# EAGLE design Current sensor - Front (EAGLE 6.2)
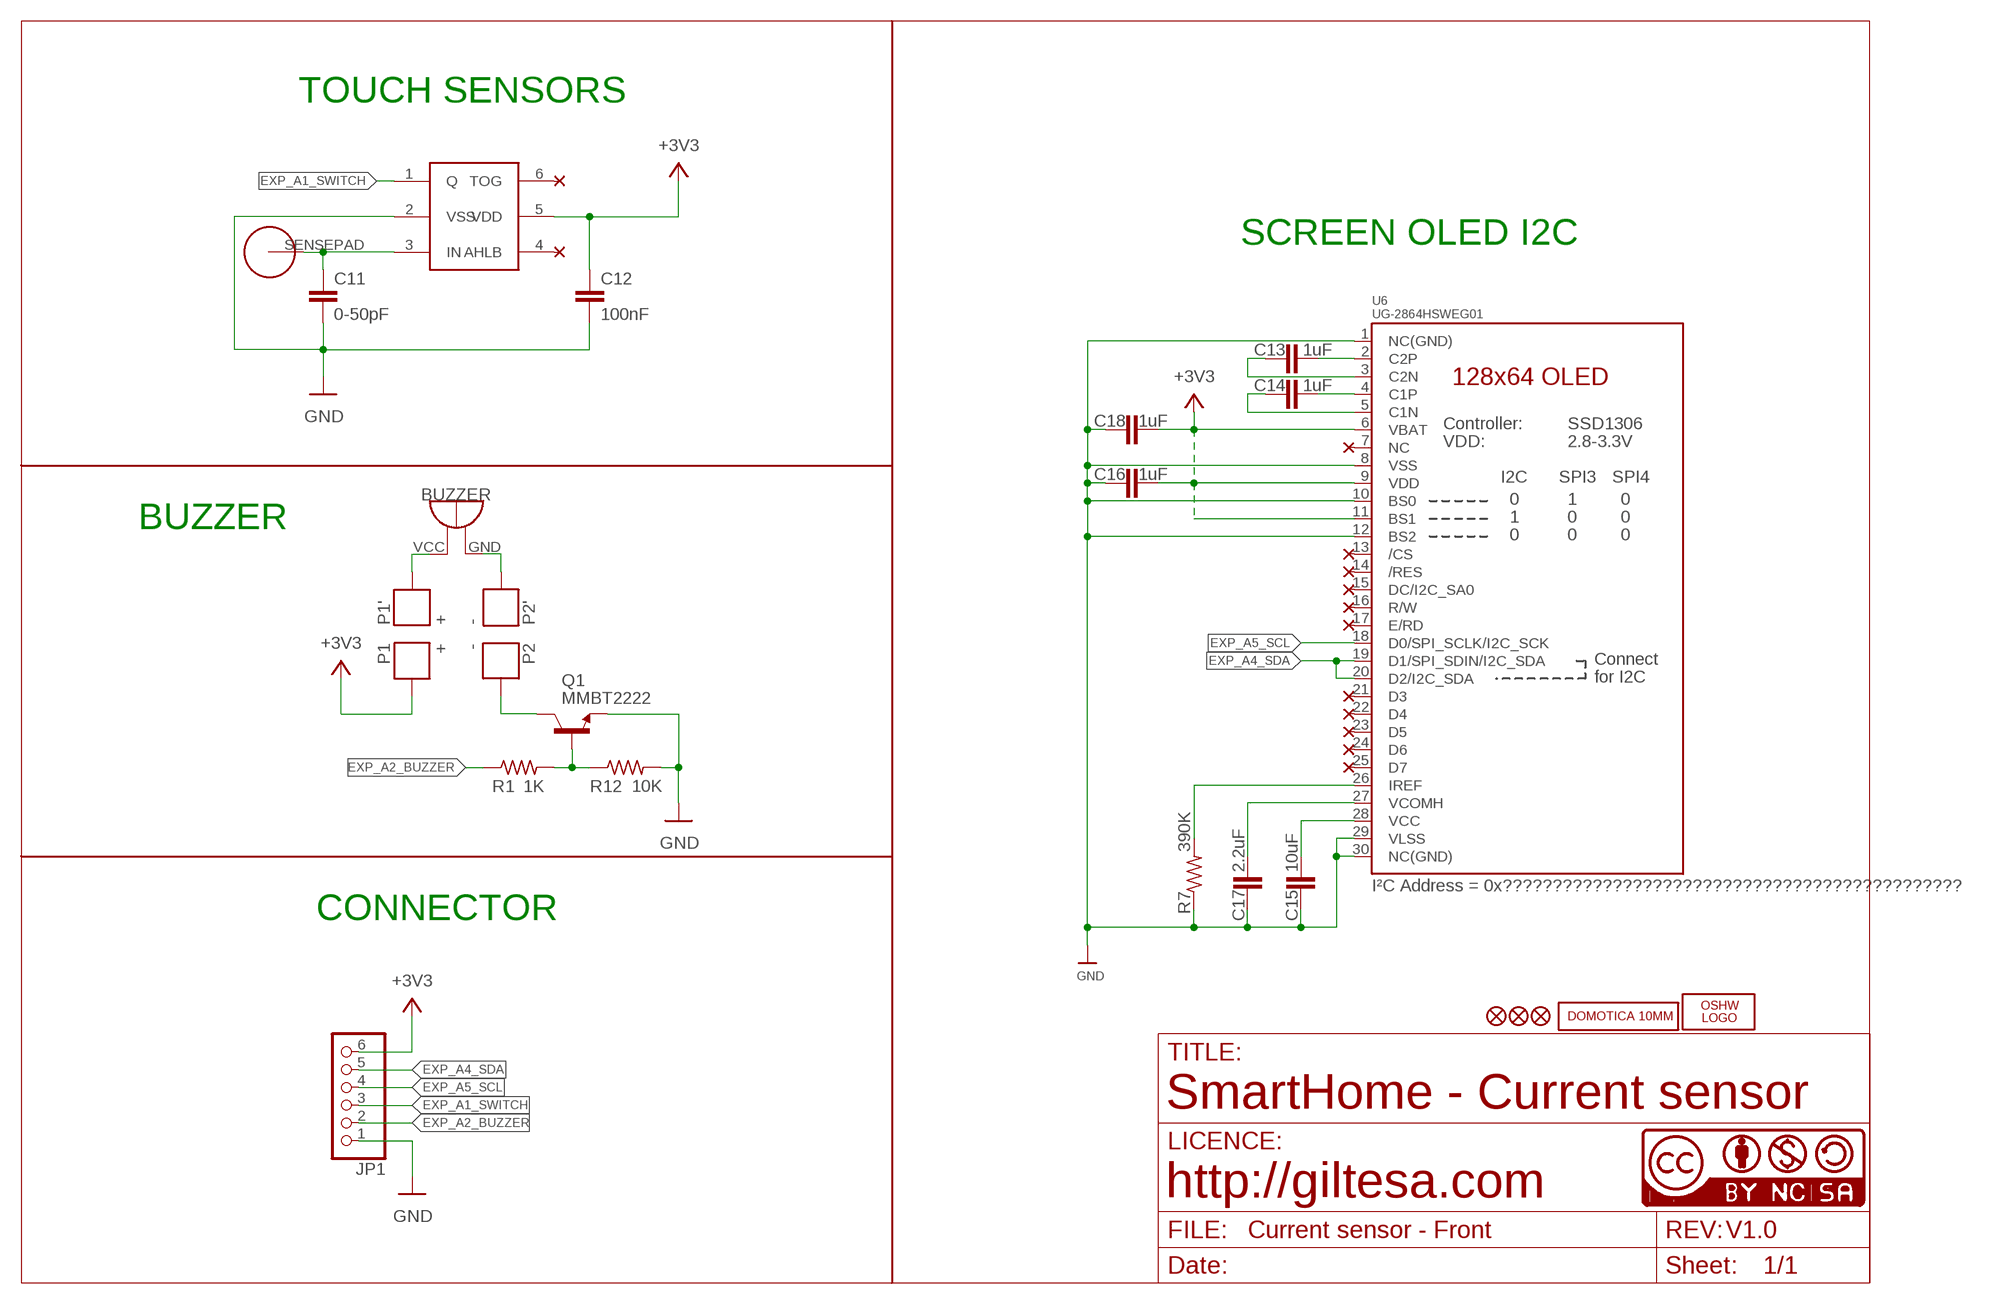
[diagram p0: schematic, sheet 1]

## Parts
BUZZER  BUZZER_9MM  [BUZZER_9MM]
C11  0-50pF  C0603  [C0603]
C12  100nF  C0603  [C0603]
C13  1uF  C0603  [C0603]
C14  1uF  C0603  [C0603]
C15  10uF  C0805  [C0805]
C16  1uF  C0603  [C0603]
C17  2.2uF  C0805  [C0805]
C18  1uF  C0603  [C0603]
JP1  PINHD-1X6B  [1X06-BIG]
LOGO1  OSHW_LOGO_FILLX0150-NT  [OSHW_FILLX150_NOTEXT]
P1  +  1X01_SMT_1.8MM  [1X01_SMT_1.8MM]
P1'  +  1X01_SMD_0.5MM  [1X01_SMD_0.5MM]
P2  -  1X01_SMT_1.8MM  [1X01_SMT_1.8MM]
P2'  -  1X01_SMD_0.5MM  [1X01_SMD_0.5MM]
Q1  MMBT2222  TRANSISTOR_NPNSOT23  [SOT23]
R1  1K  R0603  [R0603]
R7  390K  R0805  [R0805]
R12  10K  R0603  [R0603]
TTP1  TTP223  TTP223-BA6  [SOT-23-6]
U6  UG-2864HSWEG01  DISP_OLED_UG-2864HSWEG010.96"_2  [UG-2864HSWEG01_0.96IN_WRAPAROUND_2]
U$5  DOMOTICA-10MM  [DOMOTICA-10MM]
U$6  FIDUCIAL1X2  [FIDUCIAL-1X2]
U$7  FIDUCIAL1X2  [FIDUCIAL-1X2]
U$10  HTTM_SENSEPAD_NO_MARK  [HTTM_SENSEPAD_NO_MARK]
U$14  FIDUCIAL1X2  [FIDUCIAL-1X2]
U$20  CC-NC-BCNIX  [CC-NC-B_NIX]

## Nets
+3V3: C12.1 C16.2 C18.2 JP1.6 P1.P$1 TTP1.5(VDD) U6.6(VBAT) U6.9(VDD) U6.11(BS1)
EXP_A1_SWITCH: JP1.3 TTP1.1(Q)
EXP_A2_BUZZER: JP1.2 R1.1
EXP_A4_SDA: JP1.5 U6.19(D1/SPI_SDIN/I2C_SDA) U6.20(D2/I2C_SDA)
EXP_A5_SCL: JP1.4 U6.18(D0/SPI_SCLK/I2C_SCK)
GND: C11.2 C12.2 C15.1 C16.1 C17.1 C18.1 JP1.1 Q1.2(E) R7.1 R12.2 TTP1.2(VSS) U6.1(NC(GND)) U6.8(VSS) U6.10(BS0) U6.12(BS2) U6.29(VLSS) U6.30(NC(GND))
N$1: BUZZER.VCC P1'.P$1
N$2: BUZZER.GND P2'.P$1
N$3: P2.P$1 Q1.3(C)
N$6: Q1.1(B) R1.2 R12.1
N$8: C15.2 U6.28(VCC)
N$9: C17.2 U6.27(VCOMH)
N$10: C13.2 U6.2(C2P)
N$11: C13.1 U6.3(C2N)
N$13: C11.1 TTP1.3(IN) U$10.SENSEPAD
N$14: C14.2 U6.4(C1P)
N$15: C14.1 U6.5(C1N)
N$16: R7.2 U6.26(IREF)
Unconnected: TTP1.4(AHLB) TTP1.6(TOG) U6.7(NC) U6.13(/CS) U6.14(/RES) U6.15(DC/I2C_SA0) U6.16(R/W) U6.17(E/RD) U6.21(D3) U6.22(D4) U6.23(D5) U6.24(D6) U6.25(D7)

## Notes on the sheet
- TOUCH SENSORS
- SCREEN OLED I2C
- BUZZER
- I²C Address = 0x??????????????????????????????????????????????
- CONNECTOR
- SmartHome - Current sensor
- http://giltesa.com
- V1.0

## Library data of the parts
BUZZER = ,giltesa:BUZZER
C11-C14 C16 C18 = ,giltesa:C0603
C15 C17 = ,giltesa:C0805
JP1 = adafruit:PINHD-1X6: PIN HEADER
LOGO1 = ohw-logo:OSHW_LOGO_FILL
P1 P1' P2 P2' = ,giltesa:1X01
Q1 = SparkFun:TRANSISTOR_NPN: Transistor NPN BJT configuration in SOT23 package. MMBT2222 is the common NPN we use. Double check BCE configuration again layout.
R1 R12 = ,giltesa:R0603
R7 = ,giltesa:R0805
TTP1 = NCA_Sensors:TTP223-BA6: TTP223 touch sensor
U6 = microbuilder:DISP_OLED_UG-2864HSWEG01: UG-2864HSWEG01 OLED display Both 1.3" and 0.96" models share the same FPC tab footprint, only the screen dimensions vary.
U$5 = ,giltesa_logos:DOMOTICA-10MM
U$6 U$7 U$14 = SparkFun:FIDUCIAL: Fiducial Alignment Points
U$10 = ,giltesa:HTTM_SENSEPAD
U$20 = cc-by-nc-sa:CC-NC-BC: All hardware is licensed under the Creative Commons

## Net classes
2 gnd: width 0.305 mm, drill 0.406 mm, clearance 0.203 mm
3 usbvcc: width 0.203 mm, drill 0.406 mm, clearance 0.203 mm
4 USBpair: width 0.254 mm, drill 0.406 mm, clearance 0.61 mm

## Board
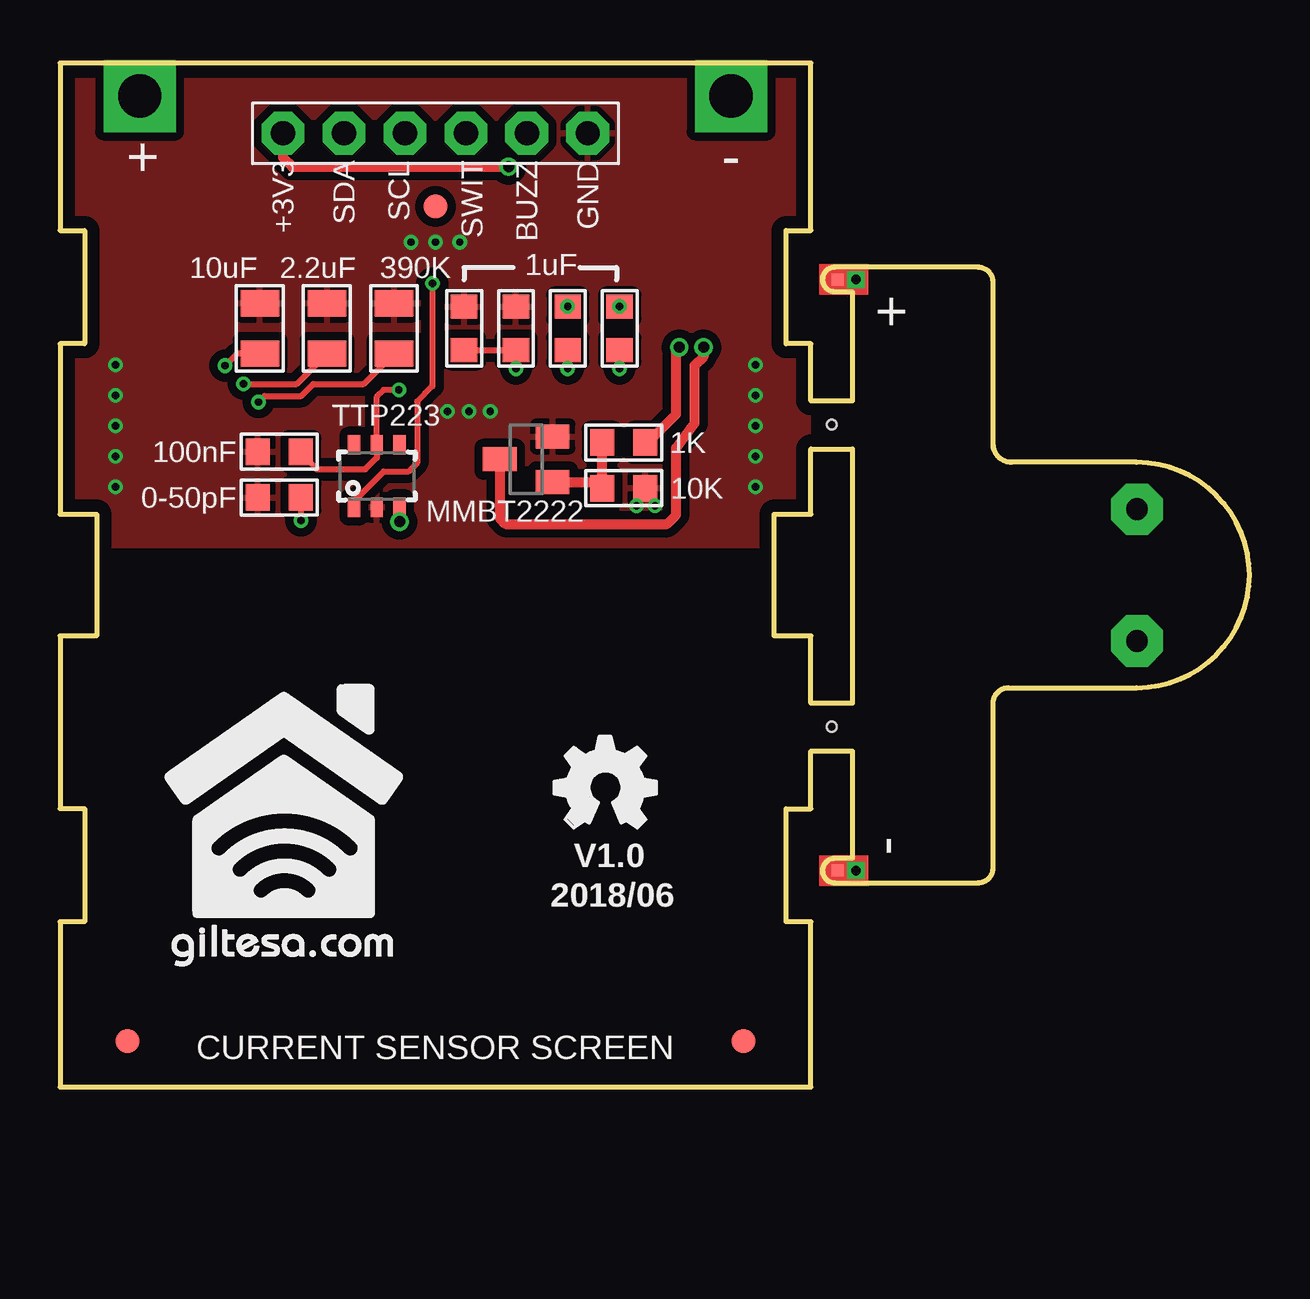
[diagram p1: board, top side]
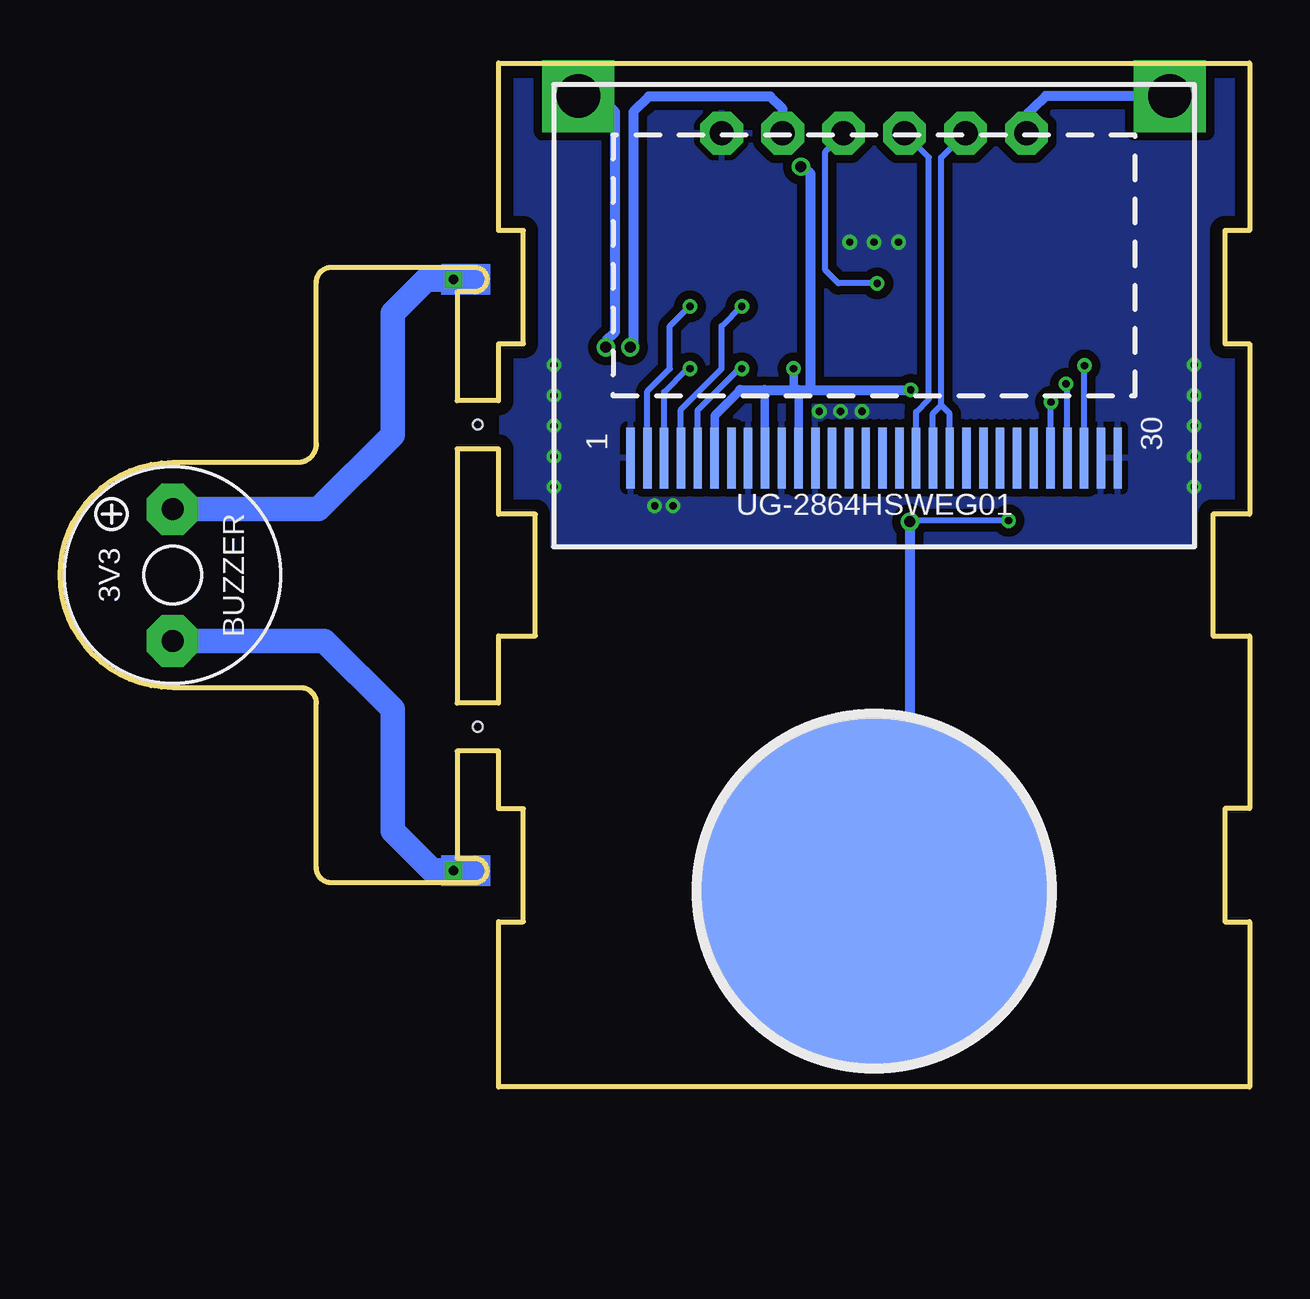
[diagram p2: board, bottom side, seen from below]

Size 49.56 x 42.67 mm. Coordinates in mm from the lower left corner, seen from the top.
Outline: 0,0 31.28,0 31.28,6.88 30.26,6.88 30.26,11.59 31.28,11.59 31.28,13.99 33.02,13.99 33.02,9.53 32.28,9.53 arc180 32.28,8.51 38.25,8.51 arc90 38.88,9.14 38.88,16 arc-90 39.52,16.64 44.86,16.64 arc180 44.86,26.04 39.64,26.04 arc-90 38.88,26.8 38.88,33.53 arc90 38.25,34.16 32.28,34.16 arc180 32.28,33.15 33.02,33.15 33.02,28.6 31.28,28.6 31.28,30.97 30.26,30.97 30.26,35.69 31.28,35.69 31.28,42.67 0,42.67 0,35.69 1.03,35.69 1.03,30.98 0,30.98 0,23.88 1.52,23.88 1.52,18.8 0,18.8 0,11.6 1.03,11.6 1.03,6.88 0,6.88 0,0
Outline: 31.28,16 31.28,18.8 29.76,18.8 29.76,23.88 31.28,23.88 31.28,26.59 33.02,26.59 33.02,16 31.28,16
Copper layers (1*16): Top 0.035mm / dielectric 1.6mm / Bottom 0.035mm
Design rules: minimum track width 6mil, minimum drill 12mil, track to track 6mil, track to pad 6mil, pad to pad 6mil, via to via 8mil, smd to smd 0mil, copper to edge 20mil, drill to drill 10mil, minimum pad ring 6mil, minimum via ring 6mil, stop-mask expansion 0mil, vias tented up to drill 100mil, thermal gap 10mil
Holes 0.41 mm at 32.15,27.61 32.15,15.01
tRestrict: area 31.6,8.1 to 33.7,34.5
bRestrict: area 31.6,8.1 to 33.7,34.5

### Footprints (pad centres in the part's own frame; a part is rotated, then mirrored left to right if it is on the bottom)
BUZZER_9MM = drill 0.914 pad 2.159 octagon: GND -2.743,0; VCC 2.743,0
C0603 = smd 1 x 1.1: 1 -0.901,0; 2 0.901,0
C0805 = smd 1.1 x 1.6: 1 -1.05,0; 2 1.05,0
1X06-BIG = drill 1.016 pad 1.778 octagon: 1 -6.35,0; 2 -3.81,0; 3 -1.27,0; 4 1.27,0; 5 3.81,0; 6 6.35,0
1X01_SMT_1.8MM = drill 1.8 pad 3 square: P$1 0,0
1X01_SMD_0.5MM = smd 0.5 x 0.5: P$1 0,0
SOT23 = smd 1 x 1.4: 1 -0.95,-1.1; 2 0.95,-1.1; 3 0,1.1
R0603 = smd 1 x 1.1: 1 -0.901,0; 2 0.901,0
R0805 = smd 1.1 x 1.6: 1 -1.05,0; 2 1.05,0
SOT-23-6 = smd 0.51 x 0.8: 1 0.955,-0.03; 2 1.905,-0.03; 3 2.855,-0.03; 4 2.855,2.57; 5 1.905,2.57; 6 0.955,2.57
UG-2864HSWEG01_0.96IN_WRAPAROUND_2 = smd 0.35 x 2.54 bottom: 1 10.15,-1.2; 2 9.45,-1.2; 3 8.75,-1.2; 4 8.05,-1.2; 5 7.35,-1.2; 6 6.65,-1.2; 7 5.95,-1.2; 8 5.25,-1.2; 9 4.55,-1.2; 10 3.85,-1.2; 11 3.15,-1.2; 12 2.45,-1.2; 13 1.75,-1.2; 14 1.05,-1.2; 15 0.35,-1.2; 16 -0.35,-1.2; 17 -1.05,-1.2; 18 -1.75,-1.2; 19 -2.45,-1.2; 20 -3.15,-1.2; 21 -3.85,-1.2; 22 -4.55,-1.2; 23 -5.25,-1.2; 24 -5.95,-1.2; 25 -6.65,-1.2; 26 -7.35,-1.2; 27 -8.05,-1.2; 28 -8.75,-1.2; 29 -9.45,-1.2; 30 -10.15,-1.2
FIDUCIAL-1X2 = smd 1 x 1: 1 0,0
HTTM_SENSEPAD_NO_MARK = smd 14.5 x 14.5: SENSEPAD -0.001,0.001

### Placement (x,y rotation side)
BUZZER  44.87,21.34 90 bottom
C11  9.14,24.57 180 top
C12  9.14,26.48 180 top
C13  23.32,31.61 90 top
C14  21.16,31.61 90 top
C15  8.33,31.61 270 top
C16  16.84,31.61 270 top
C17  11.13,31.61 270 top
C18  19,31.61 270 top
JP1  15.64,39.75 180 top
LOGO1  20.59,10.79 0 top
P1  3.32,41.3 0 top
P1'  32.41,33.66 270 top
P2  27.96,41.3 0 top
P2'  32.41,9.02 270 top
Q1  19.42,26.16 90 top
R1  23.49,26.86 180 top
R7  13.92,31.61 270 top
R12  23.49,24.95 0 top
TTP1  11.3,24.19 0 top
U6  15.64,27.42 0 top
U$5  4.34,4.95 0 top
U$6  2.81,1.91 0 top
U$7  15.64,36.7 0 top
U$10  15.64,8.16 180 bottom
U$14  28.48,1.91 0 top
U$20  0.02,0 0 top

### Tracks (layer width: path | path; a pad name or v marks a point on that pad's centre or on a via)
+3V3  (via drill 0.3, 0.46)
  Top 0.254: v18.99,29.94 C18.2 C16.2 | v14.12,29.05 13.48,29.05 13.2,28.77 TTP1.5 13.2,26.23 12.72,25.75 10.69,25.75 10.04,26.4 C12.1
  Top 0.406: JP1.6 9.29,38.73 9.67,38.35 v18.69,38.35
  Bottom 0.254: 18.79,29.03 18.82,29.05 18.94,29.05 18.99,29.1 | 20.19,28.95 20.21,29.05
  Bottom 0.356: U6.6 22.29,27.99 21.23,29.05 | U6.11 18.79,29.03 | U6.9 20.19,28.95 | v18.99,29.94 18.99,29.1
  Bottom 0.406: 21.23,29.05 20.21,29.05 18.94,29.05 | 18.82,29.05 18.31,29.05 | 18.31,29.05 v14.12,29.05 | v18.69,38.35 18.31,38.1 18.31,29.05 | P1.P$1 8.5,41.3 9.04,40.77 9.16,40.64 9.29,40.51 JP1.6
EXP_A1_SWITCH  (via drill 0.3)
  Top 0.254: TTP1.1 12.25,24.42 13.48,25.65 14.53,25.65 14.88,26 14.88,28.57 15.51,29.21 v15.51,33.5
  Bottom 0.254: JP1.3 17.67,38.99 17.67,34.04 17.13,33.5 v15.51,33.5
EXP_A2_BUZZER  (via drill 0.46)
  Top 0.406: R1.1 24.5,26.86 25.67,28.04 25.67,30.7 v25.8,30.83
  Bottom 0.406: JP1.2 19.45,40.77 19.96,41.27 25.04,41.27 25.67,40.64 25.67,30.96 v25.8,30.83
EXP_A4_SDA
  Bottom 0.254: U6.19 13.19,28.07 12.85,28.42 | U6.20 12.49,28.06 12.85,28.42 | 12.85,28.42 12.85,38.73 JP1.5
EXP_A5_SCL
  Bottom 0.254: U6.18 13.89,28.13 13.36,28.67 13.36,38.73 JP1.4
GND  (via drill 0.3)
  other vias: 2.31,30.1 2.31,28.83 2.31,27.56 2.31,26.29 2.31,25.02 28.98,30.1 28.98,28.83 28.98,27.56 28.98,26.29 28.98,25.02 24.79,24.23 24.02,24.23 15.64,35.21 14.63,35.21 16.66,35.21 17.93,28.16 17.04,28.16 16.15,28.16
  pour Bottom (isolate 0.356): 31.25,42.93 0.03,42.93 0.03,22.57 31.25,22.57
  pour Top (isolate 0.356): 31.25,42.93 0.03,42.93 0.03,22.57 31.25,22.57
N$1  (via drill 0.41)
  Top 0.406: P1'.P$1 v33.17,33.66
  Bottom 1.016: v33.17,33.66 34.31,33.66 35.71,32.26 35.71,27.18 38.81,24.08 BUZZER.VCC
N$2  (via drill 0.41)
  Top 0.406: P2'.P$1 v33.17,9.02
  Bottom 1.016: v33.17,9.02 34.06,9.02 35.71,10.67 35.71,15.75 38.55,18.59 BUZZER.GND
N$3  (via drill 0.46)
  Top 0.406: Q1.3 18.32,23.7 18.56,23.46 25.29,23.46 25.67,23.84 25.67,26.64 26.44,27.65 26.44,30.07 26.82,30.45 v26.82,30.83
  Bottom 0.406: v26.82,30.83 26.82,31.08 26.44,31.46 26.44,40.64 26.94,41.15 27.8,41.15 P2.P$1
N$6
  Top 0.406: Q1.1 22.33,25.21 R12.1 R1.2
N$8  (via drill 0.3)
  Top 0.254: C15.2 7.38,30.57 v6.88,30.07
  Bottom 0.254: U6.28 6.89,30.05 v6.88,30.07
N$9  (via drill 0.3)
  Top 0.254: v7.64,29.3 9.87,29.3 C17.2
  Bottom 0.254: U6.27 7.59,29.38 v7.64,29.3
N$10  (via drill 0.3)
  Top 0.254: v23.31,32.53 C13.2
  Bottom 0.254: U6.2 25.09,29 24.15,29.94 24.15,31.72 23.31,32.56 v23.31,32.53
N$11  (via drill 0.3)
  Top 0.254: v23.31,29.94 C13.1
  Bottom 0.254: U6.3 24.39,28.97 23.42,29.94 v23.31,29.94
N$13  (via drill 0.3, 0.46)
  Top 0.254: C11.1 v10.04,23.61 10.05,23.46
  Top 0.406: TTP1.3 v14.15,23.56
  Bottom 0.254: 14.15,11.65 U$10.SENSEPAD | v10.04,23.61 14.07,23.61 v14.15,23.56
  Bottom 0.406: v14.15,23.56 14.15,11.65
N$14  (via drill 0.3)
  Top 0.254: v21.15,32.53 C14.2
  Bottom 0.254: U6.4 23.69,28.24 21.99,29.94 21.99,31.72 21.15,32.56 v21.15,32.53
N$15  (via drill 0.3)
  Top 0.254: v21.15,29.94 C14.1
  Bottom 0.254: U6.5 22.99,28.21 21.26,29.94 v21.15,29.94
N$16  (via drill 0.3)
  Top 0.254: v8.28,28.54 8.53,28.8 10.05,28.8 10.56,29.3 12.66,29.3 R7.2
  Bottom 0.254: U6.26 8.29,28.53 v8.28,28.54
(copper drawn outside any net)
  shapes: Bottom area x2, Top area x2

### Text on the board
tPlace: +3V3 | SDA | SCL | SWIT | BUZZ | GND | V1.0 | 2018/06 | CURRENT SENSOR SCREEN
bPlace: 3V3

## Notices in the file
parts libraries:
cc-by-nc-sa: Attribution-Noncommercial-Share Alike 2.5 Switzerland License. To view a copy of this license, visit http://creativecommons.org/licenses/by-nc-sa/2.5/ch/ or send a letter to Creative Commons, 171 Second Street, Suite 300, San Francisco, California, 94105, USA.
